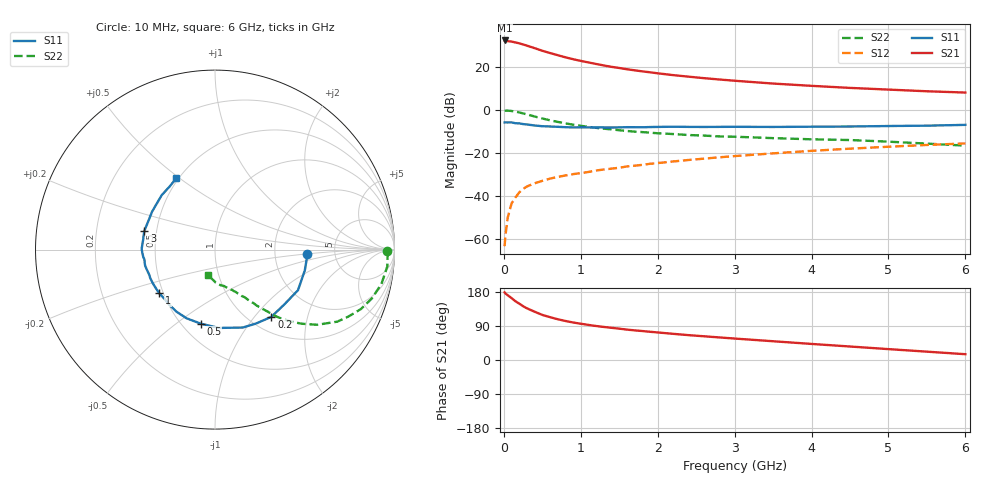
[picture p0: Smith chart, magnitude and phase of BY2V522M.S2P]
! SIEMENS Small Signal Semiconductors
! BFY420
! Si NPN RF SIEGET Grounded Emitter Transistor in MICRO-X
! VCE = 2.5 V  IC = 22 mA
! Common Emitter S-Parameters:  October  1996
# GHz  S  MA  R  50
!  f  S11  S21  S12  S22
! GHz  MAG  ANG  MAG  ANG  MAG  ANG  MAG  ANG
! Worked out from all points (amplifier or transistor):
!   36 points, 10 MHz to 6 GHz, reference 50 ohm
!   highest |S21| = 32.2 dB at 10 MHz (marker M1)
!   |S21| within 3 dB of that: start of sweep to 351.8 MHz
!   unconditionally stable (mu >= 1): 1.919 GHz to end of sweep
!   at 250 MHz: K = 0.31, MSG = 33.5 dB, |S12| = -36.6 dB
!   at 1.4 GHz: K = 0.93, MSG = 23.6 dB, |S12| = -27.2 dB
!   at 6 GHz: K = 1.07, MAG = 10.2 dB, |S12| = -15.5 dB
!   S11 on the Smith chart (normalised r, x): 10 MHz: 3.10, -0.20; 200 MHz: 1.25, -1.23; 500 MHz: 0.62, -0.62; 1 GHz: 0.47, -0.27; 3 GHz: 0.43, +0.11; 6 GHz: 0.49, +0.48
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0.01  0.5145 -2.7  40.73 178.4  0.0007 120.3  0.9594 -0.5
0.02  0.514 -5.3  40.43 175.5  0.0012 86.1  0.962 -1.8
0.1  0.5148 -26.1  38.38 163.5  0.0068 83.0  0.9468 -11.7
0.15  0.4926 -38.1  36.61 155.1  0.0093 75.0  0.9147 -17.4
0.2  0.489 -50.0  34.99 148.8  0.0123 70.9  0.8775 -22.2
0.25  0.4712 -60.8  32.92 142.0  0.0148 67.4  0.8311 -26.7
0.3  0.4611 -70.3  30.88 136.4  0.0169 67.0  0.7909 -30.5
0.4  0.4371 -87.0  27.05 127.4  0.02 62.9  0.7058 -36.4
0.5  0.4204 -100.7  23.51 119.0  0.0228 60.9  0.6344 -40.6
0.6  0.4142 -112.4  20.84 113.0  0.0257 59.8  0.5769 -43.8
0.7  0.4071 -121.6  18.57 107.6  0.0281 58.8  0.5293 -46.3
0.8  0.3994 -129.5  16.58 103.0  0.0304 57.9  0.4889 -48.3
1  0.3948 -142.0  13.69 95.7  0.0345 58.8  0.4299 -50.9
1.1  0.3935 -148.2  12.61 92.6  0.0366 59.0  0.406 -52.3
1.3  0.3943 -156.0  10.73 87.2  0.0418 58.4  0.3684 -54.2
1.6  0.3995 -166.8  8.767 80.2  0.0491 58.8  0.3259 -57.2
2.2  0.4088 179.6  6.419 69.1  0.0641 57.2  0.2769 -62.3
3  0.4072 164.9  4.751 56.6  0.0854 52.9  0.24 -68.4
3.5  0.404 156.4  4.088 49.5  0.0988 49.8  0.2226 -72.5
4.5  0.4138 141.4  3.243 35.6  0.1268 41.8  0.201 -81.1
5.5  0.4328 125.8  2.71 22.0  0.1547 32.5  0.1662 -95.0
6  0.4517 118.7  2.53 15.3  0.1679 27.8  0.1492 -104.8
